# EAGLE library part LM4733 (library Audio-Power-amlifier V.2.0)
3 Channel 30W Audio Power Amplifier with Mute
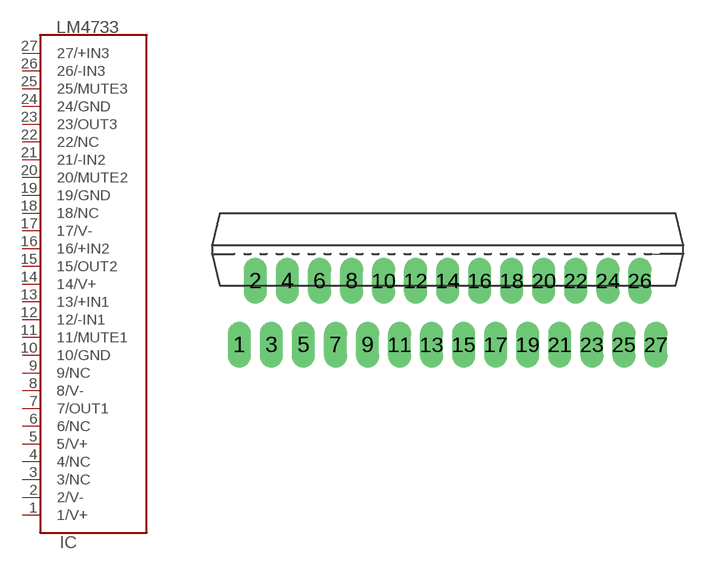
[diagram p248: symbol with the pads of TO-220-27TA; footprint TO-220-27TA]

Designator prefix IC

## LM4733  [TO-220-27TA]
1  1/V+  pwr
2  2/V-  pwr
3  3/NC  nc
4  4/NC  nc
5  5/V+  pwr
6  6/NC  nc
7  7/OUT1  out
8  8/V-  pwr
9  9/NC  nc
10  10/GND  pwr
11  11/MUTE1  in
12  12/-IN1  in
13  13/+IN1  in
14  14/V+  pwr
15  15/OUT2  out
16  16/+IN2  in
17  17/V-  out
18  18/NC  nc
19  19/GND  pwr
20  20/MUTE2  in
21  21/-IN2  in
22  22/NC  nc
23  23/OUT3  out
24  24/GND  pwr
25  25/MUTE3  in
26  26/-IN3  in
27  27/+IN3  in

## Footprint TO-220-27TA (pad centres in mm)
TO-220_MKT-TA27A , MOLDED (inch. 1,150x0,618x0,177 - body_0,040 pitch )
drill 0.5 pad 1.422 long: 1 -13.007,-3.988; 2 -12.009,0; 3 -11.008,-3.988; 4 -10.008,0; 5 -9.007,-3.988; 6 -8.006,0; 7 -7.005,-3.988; 8 -6.002,0; 9 -5.004,-3.988; 10 -4.003,0; 11 -3.002,-3.988; 12 -1.999,0; 13 -1.001,-3.99; 14 0,0; 15 1.001,-3.988; 16 2.002,0; 17 3.002,-3.988; 18 4.003,0; 19 5.004,-3.988; 20 6.007,0; 21 7.005,-3.988; 22 8.006,0; 23 9.009,-3.988; 24 10.008,0; 25 11.008,-3.988; 26 12.009,0; 27 13.01,-3.988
